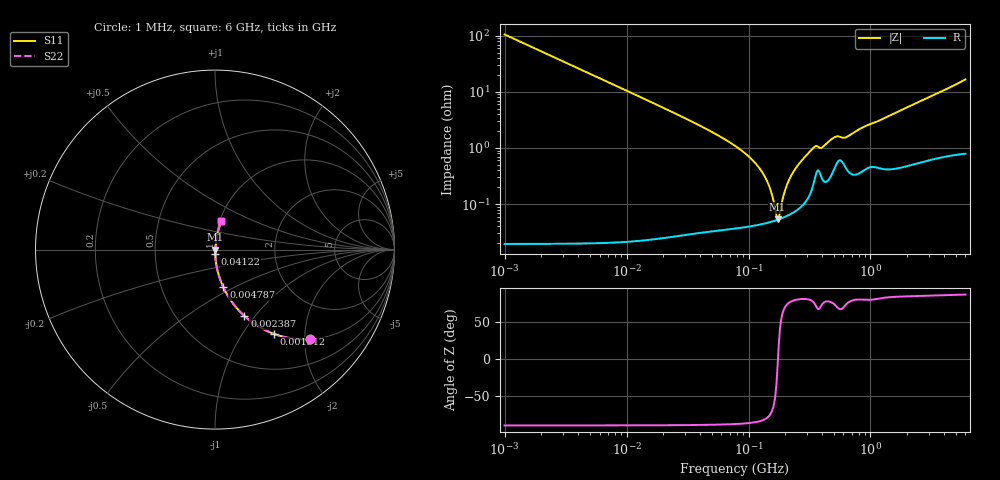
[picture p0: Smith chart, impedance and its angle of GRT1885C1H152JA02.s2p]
!Murata Part Number: GRT1885C1H152JA02
!These Parameters are Measured in Series Mode Connection
!Data Generated on Jun 19, 2026
!  o--ll--o
!Port1  Port2
!  o------o
!Operation Temp=25[degC], DC Bias Voltage=0[V]
!Freq. Start=1000[kHz] Stop=6[GHz] 401[Steps]
# Hz S RI R 50
!Freq.(Hz) S11(Real) S11(Imag) S21(Real) S21(Imag) S12(Real) S12(Imag) S22(Real) S22(Imag)
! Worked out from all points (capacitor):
!   401 points, 1 MHz to 6 GHz, reference 50 ohm
!   read as one part in series: C = 1.5 nF near 1.044 MHz
!   lowest |Z| = 53.1 mohm at 173.2 MHz (marker M1)
!   series resonance near 174.3 MHz, so ESL is about 550 pH
!   S11 on the Smith chart (normalised r, x): 1 MHz: 1.00, -2.12; 1.512 MHz: 1.00, -1.40; 2.387 MHz: 1.00, -0.89; 4.787 MHz: 1.00, -0.44; 41.22 MHz: 1.00, -0.05; 6 GHz: 1.02, +0.33
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1000000  0.528 -0.4991  0.472 0.4991  0.472 0.4991  0.528 -0.4991
1511688  0.3286 -0.4696  0.6714 0.4696  0.6714 0.4696  0.3286 -0.4696
2386795  0.1642 -0.3702  0.8358 0.3702  0.8358 0.3702  0.1642 -0.3702
4293785  0.0573 -0.232  0.9427 0.232  0.9427 0.232  0.0573 -0.232
4787042  0.0466 -0.2104  0.9534 0.2104  0.9534 0.2104  0.0466 -0.2104
1.843659e7  0.00344 -0.0565  0.9966 0.0565  0.9966 0.0565  0.00344 -0.0565
4.12249e7  0.000892 -0.0241  0.9991 0.0241  0.9991 0.0241  0.000892 -0.0241
7.745967e7  0.000485 -0.0109  0.9995 0.0109  0.9995 0.0109  0.000485 -0.0109
1.050294e8  0.000444 -0.00641  0.9996 0.00641  0.9996 0.00641  0.000444 -0.00641
1.305463e8  0.000454 -0.00357  0.9995 0.00357  0.9995 0.00357  0.000454 -0.00357
1.487431e8  0.000478 -0.00194  0.9995 0.00194  0.9995 0.00194  0.000478 -0.00194
1.658303e8  0.000509 -0.000611  0.9995 0.000611  0.9995 0.000611  0.000509 -0.000611
1.732027e8  0.000525 -7.8e-05  0.9995 7.8e-05  0.9995 7.8e-05  0.000525 -7.8e-05
1.809028e8  0.000543 0.000456  0.9995 -0.000456  0.9995 -0.000456  0.000543 0.000456
2.016844e8  0.000602 0.00181  0.9994 -0.00181  0.9994 -0.00181  0.000602 0.00181
2.248532e8  0.000684 0.0032  0.9993 -0.0032  0.9993 -0.0032  0.000684 0.0032
3.325952e8  0.00198 0.00934  0.998 -0.00934  0.998 -0.00934  0.00198 0.00934
4.045054e8  0.00282 0.00995  0.9972 -0.00995  0.9972 -0.00995  0.00282 0.00995
5.138348e8  0.00484 0.015  0.9952 -0.015  0.9952 -0.015  0.00484 0.015
6.386712e8  0.00436 0.0151  0.9956 -0.0151  0.9956 -0.0151  0.00436 0.0151
1.428092e9  0.00551 0.037  0.9945 -0.037  0.9945 -0.037  0.00551 0.037
6e9  0.0344 0.16  0.9656 -0.16  0.9656 -0.16  0.0344 0.16
